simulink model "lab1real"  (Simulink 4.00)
settings: Solver=ode45  SolverMode=SingleTasking  StartTime=0.0  StopTime=12  FixedStep=0.001  RelTol=1e-3
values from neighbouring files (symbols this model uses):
  Convert = Convert_vec(i)    [initthrottle.m]
  Convert2 = 1.95    [initthrottle.m]
  dzpos = dzpos_vec(i)    [initthrottle.m]
  h = 0.01    [initthrottle.m]
  lK = lK'    [initthrottle.m]
  lLc = 0.1    [initthrottle.m]
  lLe = place(lphie,lgame,roots(pd))    [initthrottle.m]
  Lower = Lower_vec(i)    [initthrottle.m]
  Offset = -4.7181    [initthrottle.m]
  overlap = 2    [initthrottle.m]
  tl = tl_vec(i)    [initthrottle.m]
  TR = 100    [initthrottle.m]
  tu = tu_vec(i)    [initthrottle.m]
  uK = uK'    [initthrottle.m]
  uLc = 0.1    [initthrottle.m]
  uLe = place(uphie,ugame,roots(pd))    [initthrottle.m]
undefined symbols (not defined in the file or in its folder): lC, lGAM, lPHI, uC, uGAM, uPHI
libraries: simulink3 x3, simulink_extras x1

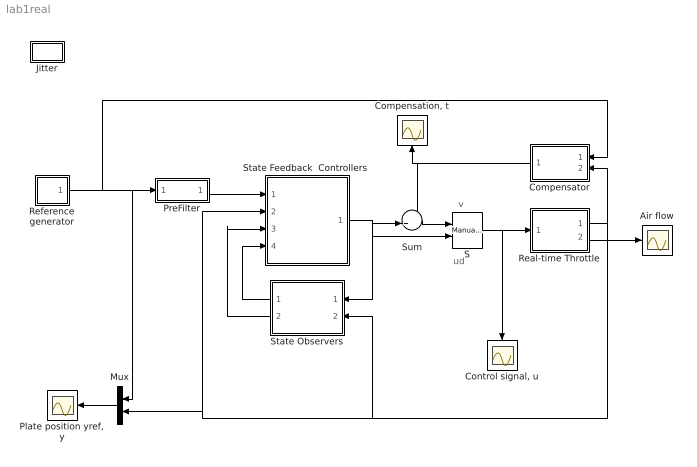
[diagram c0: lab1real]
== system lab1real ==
  note: v
  note: ud
  Air flow : Scope
  "Compensation, t" : Scope
  Compensator : Subsystem  Orientation=left
  "Control signal, u" : Scope
  Jitter : Subsystem
  Mux : Mux  Orientation=left  Inputs=2
  "Plate position yref, y" : Scope
  PreFilter : Subsystem
  Real-time Throttle : Subsystem
  Reference generator : Subsystem
  S : simulink3/Nonlinear/Manual Switch  sw=1  action=0
  "State Feedback  Controllers " : Subsystem
  State Observers : Subsystem  Orientation=left
  Sum : Sum  Inputs=++|  SaturateOnIntegerOverflow=on
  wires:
  State Observers/1(Lower xhat) -> "State Feedback  Controllers "/4(Lower xhat)
  State Observers/2(Upper xhat) -> "State Feedback  Controllers "/3(Upper xhat)
  Sum/1 -> S/1
  "State Feedback  Controllers "/1(ud) -> Sum/2, S/2, State Observers/1(ud)
  Real-time Throttle/1(y_pos) -> Mux/2, "State Feedback  Controllers "/2(y), State Observers/2(y), Compensator/2(y)
  Compensator/1(t) -> Sum/1, "Compensation, t"/1
  Mux/1 -> "Plate position yref, y"/1
  Reference generator/1(r) -> Compensator/1(ref. value), PreFilter/1(r), Mux/1
  S/1 -> "Control signal, u"/1, Real-time Throttle/1(u)
  PreFilter/1(rfiltered) -> "State Feedback  Controllers "/1(yref)
  Real-time Throttle/2(y_air) -> Air flow/1

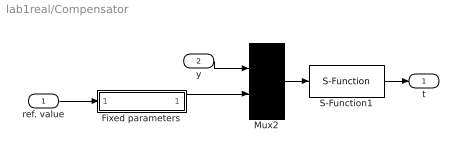
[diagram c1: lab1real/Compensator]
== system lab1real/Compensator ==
  ref. value : Inport  Port=1  LatchInput=off
  y : Inport  Port=2  LatchInput=off
  Fixed parameters : Subsystem
  Mux2 : Mux  Inputs=2
  S-Function1 : S-Function  FunctionName=compensator  Parameters=h overlap/2 -overlap/2  PortCounts=[]  SFunctionModules=''
  t : Outport  Port=1
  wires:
  Fixed parameters/1(params) -> Mux2/2
  ref. value/1 -> Fixed parameters/1(ref value)
  y/1 -> Mux2/1
  S-Function1/1 -> t/1
  Mux2/1 -> S-Function1/1

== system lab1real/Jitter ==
  Jitter plot : Scope
  S-Function1 : S-Function  FunctionName=realtimer  Parameters=h  PortCounts=[]  SFunctionModules=''
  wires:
  S-Function1/1 -> Jitter plot/1

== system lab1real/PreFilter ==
  r : Inport  Port=1  LatchInput=off
  Prefilter (with initial outputs=0) : simulink_extras/Additional Discrete/Discrete Transfer Fcn (with initial outputs)  N=[21.3 1 -20.3]  D=[835 -1596 763]  U0=[dzpos]  Y0=dzpos  TS=h
  rfiltered : Outport  Port=1
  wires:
  Prefilter (with initial outputs=0)/1 -> rfiltered/1
  r/1 -> Prefilter (with initial outputs=0)/1

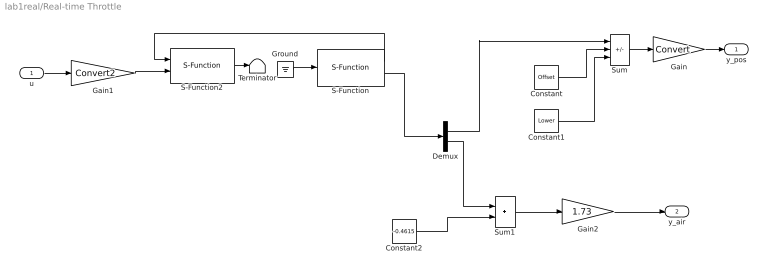
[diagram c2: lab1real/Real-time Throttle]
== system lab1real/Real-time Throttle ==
  u : Inport  Port=1  LatchInput=off
  Constant : Constant  Value=Offset
  Constant1 : Constant  Value=Lower
  Constant2 : Constant  Value=-0.4615
  Demux : Demux  Outputs=2  BusSelectionMode=off
  Gain : Gain  Gain=Convert  Multiplication=Element-wise(K.*u)  SaturateOnIntegerOverflow=on
  Gain1 : Gain  Gain=Convert2  Multiplication=Element-wise(K.*u)  SaturateOnIntegerOverflow=on
  Gain2 : Gain  Gain=1.73  Multiplication=Element-wise(K.*u)  SaturateOnIntegerOverflow=on
  Ground : Ground
  S-Function : S-Function  FunctionName=analogin  Parameters=h [0 1]  PortCounts=[]  SFunctionModules=''
  S-Function2 : S-Function  FunctionName=analogout  Parameters=h [0]  PortCounts=[]  SFunctionModules=''
  Sum : Sum  Inputs=+--  SaturateOnIntegerOverflow=on
  Sum1 : Sum  Inputs=++  SaturateOnIntegerOverflow=on
  Terminator : Terminator
  y_pos : Outport  Port=1
  y_air : Outport  Port=2
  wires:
  Gain/1 -> y_pos/1
  Ground/1 -> S-Function/1
  S-Function2/1 -> Terminator/1
  S-Function/1 -> S-Function2/1
  Constant/1 -> Sum/2
  Constant1/1 -> Sum/3
  Sum/1 -> Gain/1
  u/1 -> Gain1/1
  Gain1/1 -> S-Function2/2
  S-Function/2 -> Demux/1
  Demux/1 -> Sum/1
  Demux/2 -> Sum1/1
  Constant2/1 -> Sum1/2
  Sum1/1 -> Gain2/1
  Gain2/1 -> y_air/1

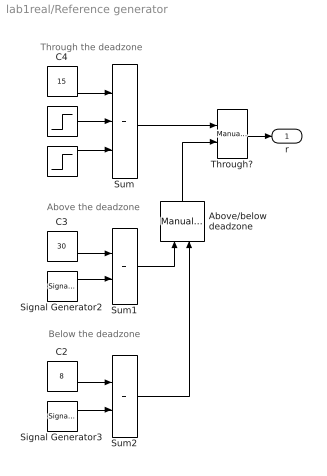
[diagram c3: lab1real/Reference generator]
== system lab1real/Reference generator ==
  note: Through the deadzone
  note: Above the deadzone
  note: Below the deadzone
  " " : Step  Time=8  Before=0  After=-6  SampleTime=0
  "  " : Step  Time=4  Before=0  After=6  SampleTime=0
  Above/below deadzone : simulink3/Nonlinear/Manual Switch  Orientation=up  sw=1  action=0
  C2 : Constant  Value=8
  C3 : Constant  Value=30
  C4 : Constant  Value=15
  Signal Generator2 : SignalGenerator  WaveForm=square  Amplitude=-5  Frequency=0.125  Units=Hertz
  Signal Generator3 : SignalGenerator  WaveForm=square  Amplitude=5  Frequency=0.125  Units=Hertz
  Sum : Sum  Inputs=+++  SaturateOnIntegerOverflow=on
  Sum1 : Sum  Inputs=++  SaturateOnIntegerOverflow=on
  Sum2 : Sum  Inputs=++  SaturateOnIntegerOverflow=on
  Through? : simulink3/Nonlinear/Manual Switch  sw=0  action=0
  r : Outport  Port=1
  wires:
  C4/1 -> Sum/1
  " "/1 -> Sum/2
  "  "/1 -> Sum/3
  Signal Generator2/1 -> Sum1/2
  C3/1 -> Sum1/1
  C2/1 -> Sum2/1
  Signal Generator3/1 -> Sum2/2
  Through?/1 -> r/1
  Sum/1 -> Through?/1
  Sum1/1 -> Above/below deadzone/1
  Sum2/1 -> Above/below deadzone/2
  Above/below deadzone/1 -> Through?/2

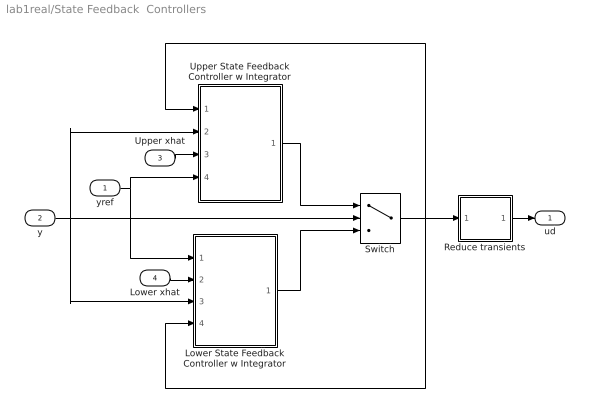
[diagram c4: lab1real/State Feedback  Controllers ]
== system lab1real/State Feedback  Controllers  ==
  yref : Inport  Port=1  LatchInput=off
  y : Inport  Port=2  LatchInput=off
  Upper xhat : Inport  Port=3  LatchInput=off
  Lower xhat : Inport  Port=4  LatchInput=off
  Lower State Feedback Controller w Integrator : Subsystem
  Reduce transients : Subsystem
  Switch : Switch  Threshold=dzpos
  Upper State Feedback Controller w Integrator : Subsystem
  ud : Outport  Port=1
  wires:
  Lower State Feedback Controller w Integrator/1(ud) -> Switch/3
  Upper State Feedback Controller w Integrator/1(ud) -> Switch/1
  Lower xhat/1 -> Lower State Feedback Controller w Integrator/2(xhat)
  Switch/1 -> Lower State Feedback Controller w Integrator/4(actual ud), Reduce transients/1(in), Upper State Feedback Controller w Integrator/1(actual ud)
  Reduce transients/1(out) -> ud/1
  Upper xhat/1 -> Upper State Feedback Controller w Integrator/3(xhat)
  y/1 -> Switch/2, Upper State Feedback Controller w Integrator/2(y), Lower State Feedback Controller w Integrator/3(y)
  yref/1 -> Upper State Feedback Controller w Integrator/4(yref), Lower State Feedback Controller w Integrator/1(yref)

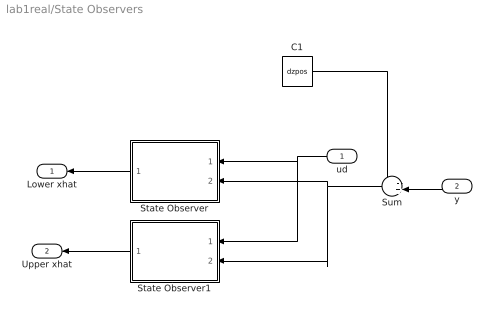
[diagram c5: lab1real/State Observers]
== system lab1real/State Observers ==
  ud : Inport  Orientation=left  Port=1  LatchInput=off
  y : Inport  Orientation=left  Port=2  LatchInput=off
  C1 : Constant  Value=dzpos
  State Observer : Subsystem  Orientation=left
  State Observer1 : Subsystem  Orientation=left
  Sum : Sum  Orientation=left  Inputs=-+|  SaturateOnIntegerOverflow=on
  Lower xhat : Outport  Orientation=left  Port=1
  Upper xhat : Outport  Orientation=left  Port=2
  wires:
  State Observer/1(xhat) -> Lower xhat/1
  ud/1 -> State Observer/1(u), State Observer1/1(u)
  y/1 -> Sum/2
  Sum/1 -> State Observer/2(y), State Observer1/2(y)
  C1/1 -> Sum/1
  State Observer1/1(xhat) -> Upper xhat/1

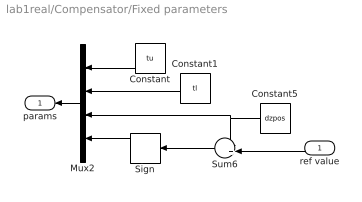
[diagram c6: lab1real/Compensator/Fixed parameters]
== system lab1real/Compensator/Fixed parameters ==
  ref value : Inport  Orientation=left  Port=1  LatchInput=off
  Constant : Constant  Orientation=left  Value=tu
  Constant1 : Constant  Orientation=left  Value=tl
  Constant5 : Constant  Orientation=left  Value=dzpos
  Mux2 : Mux  Orientation=left  Inputs=4
  Sign : Signum  Orientation=left
  Sum6 : Sum  Orientation=left  Inputs=-+|  SaturateOnIntegerOverflow=on
  params : Outport  Orientation=left  Port=1
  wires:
  Mux2/1 -> params/1
  Constant1/1 -> Mux2/2
  Sum6/1 -> Sign/1
  ref value/1 -> Sum6/2
  Constant5/1 -> Sum6/1, Mux2/3
  Constant/1 -> Mux2/1
  Sign/1 -> Mux2/4

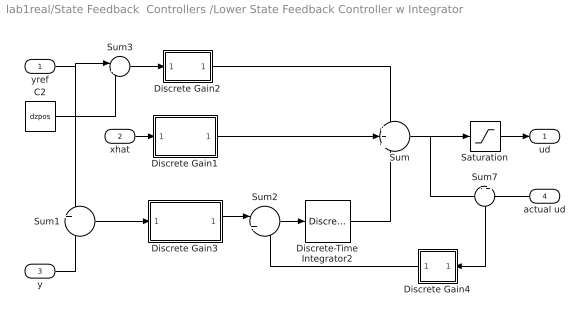
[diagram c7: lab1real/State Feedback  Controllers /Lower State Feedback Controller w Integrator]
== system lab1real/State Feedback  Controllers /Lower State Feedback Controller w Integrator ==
  yref : Inport  Port=1  LatchInput=off
  xhat : Inport  Port=2  LatchInput=off
  y : Inport  Port=3  LatchInput=off
  actual ud : Inport  Orientation=left  Port=4  LatchInput=off
  C2 : Constant  Value=dzpos
  Discrete Gain1 : Subsystem  mask(Discrete Gain){h=h, K=-lLe(1:3)}
      mask prompts: h "Sample Time"; K "Gain"
      mask init:
      | s = get_param(gcb,'MaskValueString');
      | s = s(findstr(s,'|')+1:end);
  Discrete Gain2 : Subsystem  mask(Discrete Gain){h=h, K=lLc}
      mask prompts: h "Sample Time"; K "Gain"
      mask init:
      | s = get_param(gcb,'MaskValueString');
      | s = s(findstr(s,'|')+1:end);
  Discrete Gain3 : Subsystem  mask(Discrete Gain){h=h, K=-lLe(4)}
      mask prompts: h "Sample Time"; K "Gain"
      mask init:
      | s = get_param(gcb,'MaskValueString');
      | s = s(findstr(s,'|')+1:end);
  Discrete Gain4 : Subsystem  Orientation=left  mask(Discrete Gain){h=h, K=TR}
      mask prompts: h "Sample Time"; K "Gain"
      mask init:
      | s = get_param(gcb,'MaskValueString');
      | s = s(findstr(s,'|')+1:end);
  Discrete-Time Integrator2 : DiscreteIntegrator  IntegratorMethod=ForwardEuler  ExternalReset=none  InitialConditionSource=internal  InitialCondition=0  LimitOutput=off  UpperSaturationLimit=inf  LowerSaturationLimit=-inf  ShowSaturationPort=off  ShowStatePort=off  SampleTime=h
  Saturation : Saturate  UpperLimit=7  LowerLimit=-7  LinearizeAsGain=on
  Sum : Sum  Inputs=+++  SaturateOnIntegerOverflow=on
  Sum1 : Sum  Inputs=+-  SaturateOnIntegerOverflow=on
  Sum2 : Sum  Inputs=|++  SaturateOnIntegerOverflow=on
  Sum3 : Sum  Inputs=|+-  SaturateOnIntegerOverflow=on
  Sum7 : Sum  Orientation=down  Inputs=-+  SaturateOnIntegerOverflow=on
  ud : Outport  Port=1
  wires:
  Discrete Gain2/1(Out1) -> Sum/1
  xhat/1 -> Discrete Gain1/1(In1)
  Discrete Gain1/1(Out1) -> Sum/2
  Sum7/1 -> Discrete Gain4/1(In1)
  actual ud/1 -> Sum7/2
  Sum/1 -> Sum7/1, Saturation/1
  Saturation/1 -> ud/1
  Discrete-Time Integrator2/1 -> Sum/3
  Discrete Gain3/1(Out1) -> Sum2/1
  Sum2/1 -> Discrete-Time Integrator2/1
  y/1 -> Sum1/2
  Sum1/1 -> Discrete Gain3/1(In1)
  Discrete Gain4/1(Out1) -> Sum2/2
  Sum3/1 -> Discrete Gain2/1(In1)
  yref/1 -> Sum1/1, Sum3/1
  C2/1 -> Sum3/2

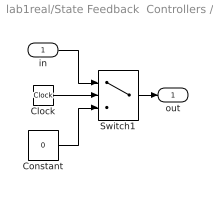
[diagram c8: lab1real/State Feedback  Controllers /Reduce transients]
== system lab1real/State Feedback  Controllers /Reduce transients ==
  in : Inport  Port=1  LatchInput=off
  Clock : Clock
  Constant : Constant  Value=0
  Switch1 : Switch  Threshold=0.03
  out : Outport  Port=1
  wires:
  Clock/1 -> Switch1/2
  in/1 -> Switch1/1
  Switch1/1 -> out/1
  Constant/1 -> Switch1/3

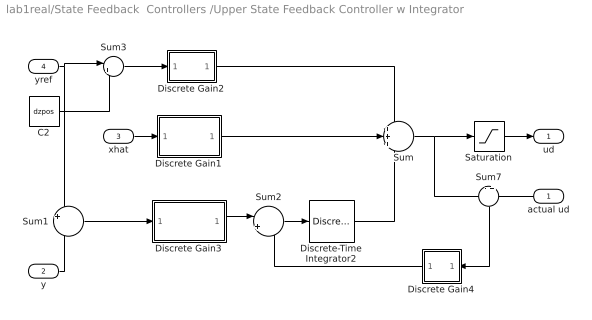
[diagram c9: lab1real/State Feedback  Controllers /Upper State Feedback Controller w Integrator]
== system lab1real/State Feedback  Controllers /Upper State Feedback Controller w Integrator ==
  actual ud : Inport  Orientation=left  Port=1  LatchInput=off
  y : Inport  Port=2  LatchInput=off
  xhat : Inport  Port=3  LatchInput=off
  yref : Inport  Port=4  LatchInput=off
  C2 : Constant  Value=dzpos
  Discrete Gain1 : Subsystem  mask(Discrete Gain){h=h, K=-uLe(1:3)}
      mask prompts: h "Sample Time"; K "Gain"
      mask init:
      | s = get_param(gcb,'MaskValueString');
      | s = s(findstr(s,'|')+1:end);
  Discrete Gain2 : Subsystem  mask(Discrete Gain){h=h, K=uLc}
      mask prompts: h "Sample Time"; K "Gain"
      mask init:
      | s = get_param(gcb,'MaskValueString');
      | s = s(findstr(s,'|')+1:end);
  Discrete Gain3 : Subsystem  mask(Discrete Gain){h=h, K=-uLe(4)}
      mask prompts: h "Sample Time"; K "Gain"
      mask init:
      | s = get_param(gcb,'MaskValueString');
      | s = s(findstr(s,'|')+1:end);
  Discrete Gain4 : Subsystem  Orientation=left  mask(Discrete Gain){h=h, K=TR}
      mask prompts: h "Sample Time"; K "Gain"
      mask init:
      | s = get_param(gcb,'MaskValueString');
      | s = s(findstr(s,'|')+1:end);
  Discrete-Time Integrator2 : DiscreteIntegrator  IntegratorMethod=ForwardEuler  ExternalReset=none  InitialConditionSource=internal  InitialCondition=0  LimitOutput=off  UpperSaturationLimit=inf  LowerSaturationLimit=-inf  ShowSaturationPort=off  ShowStatePort=off  SampleTime=h
  Saturation : Saturate  UpperLimit=7  LowerLimit=-7  LinearizeAsGain=on
  Sum : Sum  Inputs=+++  SaturateOnIntegerOverflow=on
  Sum1 : Sum  Inputs=+-  SaturateOnIntegerOverflow=on
  Sum2 : Sum  Inputs=|++  SaturateOnIntegerOverflow=on
  Sum3 : Sum  Inputs=|+-  SaturateOnIntegerOverflow=on
  Sum7 : Sum  Orientation=down  Inputs=-+  SaturateOnIntegerOverflow=on
  ud : Outport  Port=1
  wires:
  xhat/1 -> Discrete Gain1/1(In1)
  Sum7/1 -> Discrete Gain4/1(In1)
  actual ud/1 -> Sum7/2
  Sum/1 -> Sum7/1, Saturation/1
  Saturation/1 -> ud/1
  Discrete Gain3/1(Out1) -> Sum2/1
  Sum2/1 -> Discrete-Time Integrator2/1
  y/1 -> Sum1/2
  Sum1/1 -> Discrete Gain3/1(In1)
  Discrete Gain4/1(Out1) -> Sum2/2
  Discrete-Time Integrator2/1 -> Sum/3
  Discrete Gain2/1(Out1) -> Sum/1
  Discrete Gain1/1(Out1) -> Sum/2
  Sum3/1 -> Discrete Gain2/1(In1)
  yref/1 -> Sum1/1, Sum3/1
  C2/1 -> Sum3/2

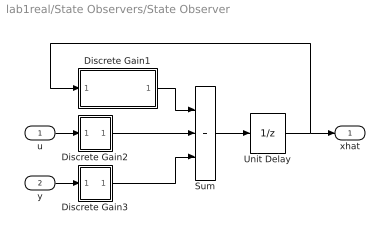
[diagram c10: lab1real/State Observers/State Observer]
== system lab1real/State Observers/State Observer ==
  u : Inport  Port=1  LatchInput=off
  y : Inport  Port=2  LatchInput=off
  Discrete Gain1 : Subsystem  mask(Discrete Gain){h=h, K=lPHI-lK*lC}
      mask prompts: h "Sample Time"; K "Gain"
      mask init:
      | s = get_param(gcb,'MaskValueString');
      | s = s(findstr(s,'|')+1:end);
  Discrete Gain2 : Subsystem  mask(Discrete Gain){h=h, K=lGAM}
      mask prompts: h "Sample Time"; K "Gain"
      mask init:
      | s = get_param(gcb,'MaskValueString');
      | s = s(findstr(s,'|')+1:end);
  Discrete Gain3 : Subsystem  mask(Discrete Gain){h=h, K=lK}
      mask prompts: h "Sample Time"; K "Gain"
      mask init:
      | s = get_param(gcb,'MaskValueString');
      | s = s(findstr(s,'|')+1:end);
  Sum : Sum  Inputs=+++  SaturateOnIntegerOverflow=on
  Unit Delay : UnitDelay  X0=0  SampleTime=h
  xhat : Outport  Port=1
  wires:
  Discrete Gain1/1(Out1) -> Sum/1
  Discrete Gain2/1(Out1) -> Sum/2
  Discrete Gain3/1(Out1) -> Sum/3
  Sum/1 -> Unit Delay/1
  Unit Delay/1 -> Discrete Gain1/1(In1), xhat/1
  u/1 -> Discrete Gain2/1(In1)
  y/1 -> Discrete Gain3/1(In1)

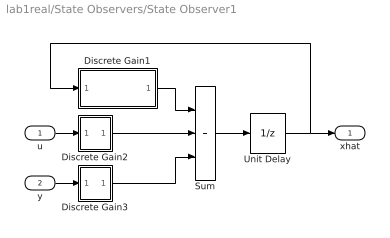
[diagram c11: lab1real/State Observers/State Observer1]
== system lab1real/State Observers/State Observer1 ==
  u : Inport  Port=1  LatchInput=off
  y : Inport  Port=2  LatchInput=off
  Discrete Gain1 : Subsystem  mask(Discrete Gain){h=h, K=uPHI-uK*uC}
      mask prompts: h "Sample Time"; K "Gain"
      mask init:
      | s = get_param(gcb,'MaskValueString');
      | s = s(findstr(s,'|')+1:end);
  Discrete Gain2 : Subsystem  mask(Discrete Gain){h=h, K=uGAM}
      mask prompts: h "Sample Time"; K "Gain"
      mask init:
      | s = get_param(gcb,'MaskValueString');
      | s = s(findstr(s,'|')+1:end);
  Discrete Gain3 : Subsystem  mask(Discrete Gain){h=h, K=uK}
      mask prompts: h "Sample Time"; K "Gain"
      mask init:
      | s = get_param(gcb,'MaskValueString');
      | s = s(findstr(s,'|')+1:end);
  Sum : Sum  Inputs=+++  SaturateOnIntegerOverflow=on
  Unit Delay : UnitDelay  X0=0  SampleTime=h
  xhat : Outport  Port=1
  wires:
  Discrete Gain1/1(Out1) -> Sum/1
  Discrete Gain2/1(Out1) -> Sum/2
  Discrete Gain3/1(Out1) -> Sum/3
  Sum/1 -> Unit Delay/1
  Unit Delay/1 -> Discrete Gain1/1(In1), xhat/1
  u/1 -> Discrete Gain2/1(In1)
  y/1 -> Discrete Gain3/1(In1)

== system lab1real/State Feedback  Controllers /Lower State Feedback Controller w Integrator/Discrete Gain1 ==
  In1 : Inport  Port=1  LatchInput=off
  Discrete State-Space : DiscreteStateSpace  A=0  B=zeros(1,size(K,2))  C=zeros(size(K,1),1)  D=K  X0=0  SampleTime=h  Realization=auto
  Out1 : Outport  Port=1
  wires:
  Discrete State-Space/1 -> Out1/1
  In1/1 -> Discrete State-Space/1

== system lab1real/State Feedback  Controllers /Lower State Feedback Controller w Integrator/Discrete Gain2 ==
  In1 : Inport  Port=1  LatchInput=off
  Discrete State-Space : DiscreteStateSpace  A=0  B=zeros(1,size(K,2))  C=zeros(size(K,1),1)  D=K  X0=0  SampleTime=h  Realization=auto
  Out1 : Outport  Port=1
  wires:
  Discrete State-Space/1 -> Out1/1
  In1/1 -> Discrete State-Space/1

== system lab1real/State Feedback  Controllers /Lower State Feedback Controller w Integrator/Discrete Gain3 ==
  In1 : Inport  Port=1  LatchInput=off
  Discrete State-Space : DiscreteStateSpace  A=0  B=zeros(1,size(K,2))  C=zeros(size(K,1),1)  D=K  X0=0  SampleTime=h  Realization=auto
  Out1 : Outport  Port=1
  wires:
  In1/1 -> Discrete State-Space/1
  Discrete State-Space/1 -> Out1/1

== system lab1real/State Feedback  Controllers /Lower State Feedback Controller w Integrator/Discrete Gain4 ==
  In1 : Inport  Port=1  LatchInput=off
  Discrete State-Space : DiscreteStateSpace  A=0  B=zeros(1,size(K,2))  C=zeros(size(K,1),1)  D=K  X0=0  SampleTime=h  Realization=auto
  Out1 : Outport  Port=1
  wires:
  Discrete State-Space/1 -> Out1/1
  In1/1 -> Discrete State-Space/1

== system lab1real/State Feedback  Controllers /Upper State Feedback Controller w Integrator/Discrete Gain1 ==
  In1 : Inport  Port=1  LatchInput=off
  Discrete State-Space : DiscreteStateSpace  A=0  B=zeros(1,size(K,2))  C=zeros(size(K,1),1)  D=K  X0=0  SampleTime=h  Realization=auto
  Out1 : Outport  Port=1
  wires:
  Discrete State-Space/1 -> Out1/1
  In1/1 -> Discrete State-Space/1

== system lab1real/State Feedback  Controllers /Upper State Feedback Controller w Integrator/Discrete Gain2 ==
  In1 : Inport  Port=1  LatchInput=off
  Discrete State-Space : DiscreteStateSpace  A=0  B=zeros(1,size(K,2))  C=zeros(size(K,1),1)  D=K  X0=0  SampleTime=h  Realization=auto
  Out1 : Outport  Port=1
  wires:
  Discrete State-Space/1 -> Out1/1
  In1/1 -> Discrete State-Space/1

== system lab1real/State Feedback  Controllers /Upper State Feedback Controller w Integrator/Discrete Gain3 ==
  In1 : Inport  Port=1  LatchInput=off
  Discrete State-Space : DiscreteStateSpace  A=0  B=zeros(1,size(K,2))  C=zeros(size(K,1),1)  D=K  X0=0  SampleTime=h  Realization=auto
  Out1 : Outport  Port=1
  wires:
  In1/1 -> Discrete State-Space/1
  Discrete State-Space/1 -> Out1/1

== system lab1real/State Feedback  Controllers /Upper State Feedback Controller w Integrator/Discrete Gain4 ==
  In1 : Inport  Port=1  LatchInput=off
  Discrete State-Space : DiscreteStateSpace  A=0  B=zeros(1,size(K,2))  C=zeros(size(K,1),1)  D=K  X0=0  SampleTime=h  Realization=auto
  Out1 : Outport  Port=1
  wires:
  Discrete State-Space/1 -> Out1/1
  In1/1 -> Discrete State-Space/1

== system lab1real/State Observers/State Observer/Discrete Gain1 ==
  In1 : Inport  Port=1  LatchInput=off
  Discrete State-Space : DiscreteStateSpace  A=0  B=zeros(1,size(K,2))  C=zeros(size(K,1),1)  D=K  X0=0  SampleTime=h  Realization=auto
  Out1 : Outport  Port=1
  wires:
  Discrete State-Space/1 -> Out1/1
  In1/1 -> Discrete State-Space/1

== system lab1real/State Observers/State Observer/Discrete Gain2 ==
  In1 : Inport  Port=1  LatchInput=off
  Discrete State-Space : DiscreteStateSpace  A=0  B=zeros(1,size(K,2))  C=zeros(size(K,1),1)  D=K  X0=0  SampleTime=h  Realization=auto
  Out1 : Outport  Port=1
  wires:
  In1/1 -> Discrete State-Space/1
  Discrete State-Space/1 -> Out1/1

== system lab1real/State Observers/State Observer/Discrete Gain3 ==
  In1 : Inport  Port=1  LatchInput=off
  Discrete State-Space : DiscreteStateSpace  A=0  B=zeros(1,size(K,2))  C=zeros(size(K,1),1)  D=K  X0=0  SampleTime=h  Realization=auto
  Out1 : Outport  Port=1
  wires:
  Discrete State-Space/1 -> Out1/1
  In1/1 -> Discrete State-Space/1

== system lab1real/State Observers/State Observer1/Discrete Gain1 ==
  In1 : Inport  Port=1  LatchInput=off
  Discrete State-Space : DiscreteStateSpace  A=0  B=zeros(1,size(K,2))  C=zeros(size(K,1),1)  D=K  X0=0  SampleTime=h  Realization=auto
  Out1 : Outport  Port=1
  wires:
  Discrete State-Space/1 -> Out1/1
  In1/1 -> Discrete State-Space/1

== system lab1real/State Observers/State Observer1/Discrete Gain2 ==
  In1 : Inport  Port=1  LatchInput=off
  Discrete State-Space : DiscreteStateSpace  A=0  B=zeros(1,size(K,2))  C=zeros(size(K,1),1)  D=K  X0=0  SampleTime=h  Realization=auto
  Out1 : Outport  Port=1
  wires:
  In1/1 -> Discrete State-Space/1
  Discrete State-Space/1 -> Out1/1

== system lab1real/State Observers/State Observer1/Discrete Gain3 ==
  In1 : Inport  Port=1  LatchInput=off
  Discrete State-Space : DiscreteStateSpace  A=0  B=zeros(1,size(K,2))  C=zeros(size(K,1),1)  D=K  X0=0  SampleTime=h  Realization=auto
  Out1 : Outport  Port=1
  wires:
  Discrete State-Space/1 -> Out1/1
  In1/1 -> Discrete State-Space/1
